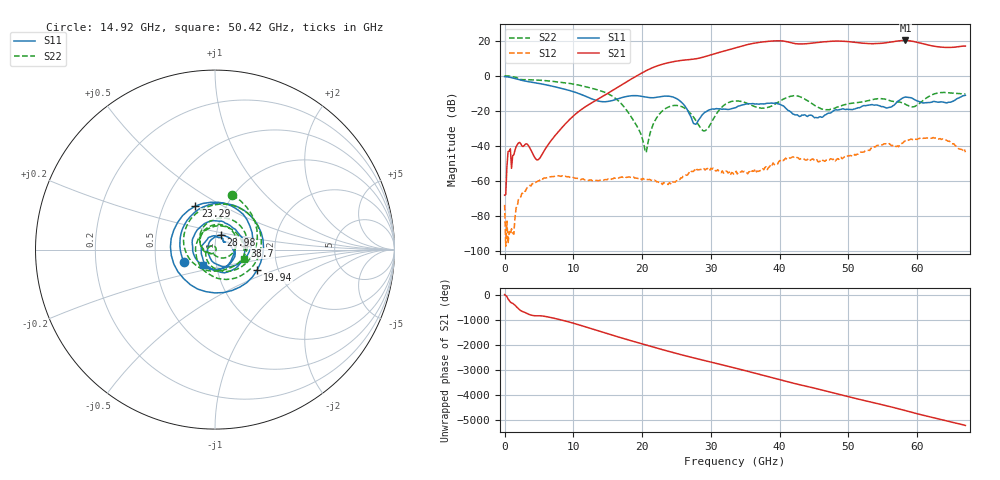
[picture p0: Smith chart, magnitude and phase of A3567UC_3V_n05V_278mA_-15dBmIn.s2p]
! MARKI MICROWAVE INC.
! Date:  4/20/2021
! Model Number:  A-3567UC
! Description:  2-port Small Signal S-parameter data for A-3567UC
! Frequency Range:  10 MHz to 67 GHz
! Port Configuration:  PORT 1: Input
!  PORT 2: Output
! Bias Condition: Vd = +3V, Vg = -0.5V, Id = 278mA
! A-3567UC s2p files are only valid for small signal conditions (below -10 dBm input power)
# Hz S  dB  R 50
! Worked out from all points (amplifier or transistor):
!   401 points, 10 MHz to 67 GHz, reference 50 ohm
!   highest |S21| = 20.2 dB at 58.29 GHz (marker M1)
!   |S21| within 3 dB of that: 34.66 GHz to 62.03 GHz (27.37 GHz wide, 56.6 % of centre)
!   unconditionally stable (mu >= 1): 185.2 MHz to end of sweep
!   at 11.06 GHz: K = 2809.06, MAG = -17.6 dB, |S12| = -59.3 dB
!   at 33.51 GHz: K = 44.44, MAG = 16.2 dB, |S12| = -55.4 dB
!   at 67 GHz: K = 8.90, MAG = 17.8 dB, |S12| = -43.5 dB
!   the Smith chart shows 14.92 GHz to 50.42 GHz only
!   S11 on the Smith chart (normalised r, x): 14.92 GHz: 0.70, -0.10; 19.94 GHz: 1.56, -0.38; 23.29 GHz: 0.72, +0.38; 28.98 GHz: 1.05, +0.17; 38.7 GHz: 1.40, +0.06; 50.42 GHz: 0.86, -0.15
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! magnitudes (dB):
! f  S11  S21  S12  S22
! 10 MHz  -0.4  -68.0  -73.6  0.0
! 679.9 MHz  -0.7  -42.9  -88.7  -0.1
! 2.02 GHz  -2.0  -38.3  -70.6  -1.6
! 4.867 GHz  -4.2  -47.8  -60.0  -2.4
! 11.23 GHz  -10.7  -19.0  -58.9  -5.6
! 14.92 GHz  -14.6  -10.2  -59.2  -9.9
! 19.94 GHz  -11.7  1.6  -59.3  -34.6
! 20.61 GHz  -12.2  3.0  -59.0  -43.7
! 22.45 GHz  -12.0  6.1  -60.8  -22.1
! 23.29 GHz  -11.5  7.0  -61.3  -18.9
! 25.63 GHz  -14.7  8.8  -58.2  -17.3
! 27.64 GHz  -27.4  9.7  -53.6  -24.4
! 28.98 GHz  -21.2  10.8  -52.9  -31.4
! 33.51 GHz  -18.1  16.0  -55.4  -14.3
! 38.7 GHz  -15.5  19.9  -50.7  -17.4
! 42.05 GHz  -21.9  18.6  -46.3  -11.3
! 44.73 GHz  -22.6  18.7  -47.4  -15.9
! 50.42 GHz  -19.2  19.4  -45.5  -15.6
! 55.95 GHz  -18.0  19.2  -38.6  -14.0
! 58.29 GHz  -12.0  20.2  -37.2  -16.2
! 63.65 GHz  -14.9  16.4  -35.9  -9.5
! 67 GHz  -11.1  17.0  -43.5  -10.4
